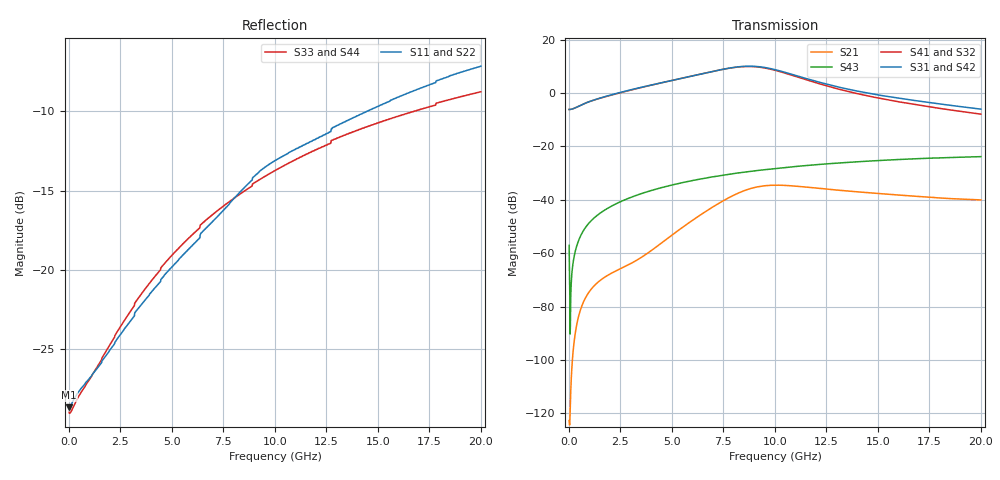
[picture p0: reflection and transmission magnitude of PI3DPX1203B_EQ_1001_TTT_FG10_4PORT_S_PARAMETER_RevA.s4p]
! NPort=4 DATA=2000 NOISE=0 GROUPDELAY=0 COMPLEX_DATAFORMAT=POLAR
! NumOfBlock=1 NumOfParam=0
! .MODEL Smodel S TSTONEFILE=PI3DPX1203B_EQ_1001_TTT_FG10_4PORT_S_PARAMETER_RevA.s4p TYPE=S
!  -- The above .MODEL line can be used for the S element in the netlist.
! The s parameter is extracted from the linear redriver, it is not bi-directional; only s(4,1)s(4,2) and s(3,1)s(3,2)
! should be the insertion loss
!Port definition:
!Port1 = input+
!Port2 = input-
!Port3 = output+
!Port4 = output-
# Hz S MA R  50
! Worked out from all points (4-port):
!   2000 points, 10 MHz to 20 GHz, reference 50 ohm
!   strongest paths, dB at 10 MHz, 5.01 GHz, 10.01 GHz, 15.01 GHz, 20 GHz:
!     S31: -6.2, 4.7, 8.7, -0.7, -6.0
!     S42: -6.2, 4.7, 8.7, -0.7, -6.0
!     S41: -6.2, 4.7, 8.5, -1.9, -7.9
!     S32: -6.2, 4.7, 8.5, -1.9, -7.9
!     S43: -57.1, -34.4, -28.3, -25.3, -23.8
!     S21: -122.7, -53.2, -34.5, -37.6, -40.0
!   lowest |S11| = -28.6 dB at 10 MHz (marker M1), VSWR 1.08, Z = 46.4 - j0.0306 ohm
!   |S11| at or under -10 dB: start of sweep to 14.49 GHz
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1e7  0.03701 -179.5  7.338e-07 10.6  0 0.0  0 0.0
     7.338e-07 10.6  0.03701 -179.5  0 0.0  0 0.0
     0.4917 -0.0  0.4917 180.0  0.03566 178.2  0.001403 -77.8
     0.4917 180.0  0.4917 -0.0  0.001403 -77.8  0.03566 178.2
3.11e9  0.07073 -126.7  0.0006748 133.5  1.612e-10 55.7  2.737e-09 107.1
        0.0006747 133.5  0.07073 -126.7  2.736e-09 107.1  1.612e-10 55.7
        1.175 -0.7  1.162 -179.5  0.0762 -126.4  0.0115 77.6
        1.162 -179.5  1.175 -0.7  0.0115 77.6  0.0762 -126.4
5.94e9  0.1186 -110.8  0.00399 151.1  1.423e-08 -120.8  1.264e-07 67.9
        0.003989 151.2  0.1186 -110.8  1.264e-07 67.9  1.423e-08 -120.8
        2.069 -41.6  2.068 140.0  0.1282 -117.1  0.02273 65.4
        2.068 140.0  2.069 -41.6  0.02273 65.4  0.1282 -117.1
8.31e9  0.176 -105.2  0.01382 110.2  3.364e-07 156.2  9.324e-07 18.9
        0.01382 110.2  0.176 -105.2  9.314e-07 18.9  3.365e-07 156.2
        3.117 -99.4  3.087 82.0  0.1735 -115.9  0.03222 53.3
        3.088 82.0  3.117 -99.4  0.03222 53.3  0.1735 -115.9
9.83e9  0.2175 -107.2  0.01874 66.6  1.13e-06 94.7  1.914e-06 -18.8
        0.01873 66.6  0.2174 -107.2  1.912e-06 -18.7  1.13e-06 94.7
        2.841 -149.1  2.769 32.1  0.2025 -116.2  0.03788 45.3
        2.771 32.1  2.84 -149.1  0.03788 45.3  0.2025 -116.2
1.204e10  0.2596 -109.2  0.01657 25.2  2.939e-06 29.4  3.67e-06 -46.9
          0.01656 25.3  0.2596 -109.1  3.67e-06 -46.8  2.941e-06 29.5
          1.638 163.4  1.535 -15.2  0.2398 -117.5  0.04559 34.0
          1.536 -15.2  1.637 163.4  0.04559 34.0  0.2398 -117.5
2e10  0.4379 -117.4  0.009912 -17.5  2.232e-05 -108.6  3.157e-05 -133.8
      0.009954 -17.4  0.438 -117.4  3.165e-05 -133.8  2.234e-05 -108.6
      0.4989 76.6  0.4024 -89.9  0.3637 -123.9  0.06431 -7.1
      0.4021 -90.1  0.4994 76.6  0.06431 -7.1  0.3637 -123.9
